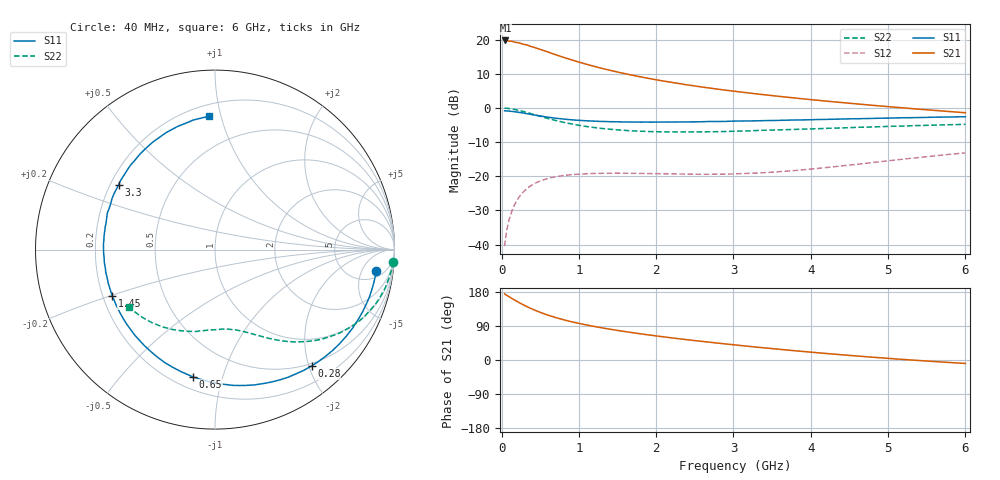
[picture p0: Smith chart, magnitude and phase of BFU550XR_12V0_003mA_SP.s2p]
! Filename:  P:\Prog\Test\Noise\ATS_data\Testdata_Net\03 Spar\BFU550XR_APG2013_45_C05_12p0V_003mA_SP_CM01_D.s2p
! Date/Time: Tue 06/Aug/2013 14:38:18
! BFU550XR_APG2013_45_C05_12p0V_1to35mA_SP_CM01_Bias3_R.s2p
! MDIF S-parameter v. bias file
! BFU550XR_APG2013_45_C05_12p0V_1to35mA_SP_CM01
! Date/time Fri Aug 02 14:58:10 2013
! VAR V_out= 12.0010
! VAR I_out= 2.9950
! VAR V_in= 0.7926
! VAR I_in= 0.0257
! Device data file deembeded for feedlines and parallel
! Original file: \03 Spar\BFU550XR_APG2013_45_C05_12p0V_003mA_SP_CM01_R.s2p
! Feed-files: PR006V01_02082013_Feed1.s2p, PR006V01_02082013_Feed2.s2p
! Parallel-file: PR006V01_02082013_Par.s2p
# MHz S MA R 50
!  Freq-MHz  S11-mag  S11-arg  S21-mag  S21-arg  S12-mag  S12-arg  S22-mag  S22-arg
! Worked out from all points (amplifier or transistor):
!   98 points, 40 MHz to 6 GHz, reference 50 ohm
!   highest |S21| = 19.7 dB at 50 MHz (marker M1)
!   |S21| within 3 dB of that: start of sweep to 552.4 MHz
!   unconditionally stable (mu >= 1): 2.794 GHz to 4.426 GHz
!   at 300 MHz: K = 0.13, MSG = 21.4 dB, |S12| = -24.2 dB
!   at 1.6 GHz: K = 0.60, MSG = 14.6 dB, |S12| = -19.1 dB
!   at 6 GHz: K = 0.81, MSG = 5.9 dB, |S12| = -13.2 dB
!   S11 on the Smith chart (normalised r, x): 40 MHz: 7, -10; 280 MHz: 0.46, -2.05; 650 MHz: 0.27, -0.80; 1.45 GHz: 0.24, -0.20; 3.3 GHz: 0.23, +0.29; 6 GHz: 0.28, +0.91
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40  0.9072 -7.6  9.7 174.6  0.009492 83.8  0.9928 -4.0
50  0.9053 -9.4  9.702 172.6  0.01185 83.3  0.9924 -5.1
120  0.8927 -22.7  9.484 164.2  0.02791 76.2  0.9725 -12.6
180  0.8762 -33.5  9.144 157.0  0.0406 70.2  0.9452 -18.6
240  0.8559 -44.0  8.877 150.1  0.05189 64.7  0.913 -24.0
280  0.8424 -50.3  8.549 145.9  0.05866 61.2  0.889 -27.4
320  0.8257 -57.2  8.391 141.7  0.0647 58.0  0.8628 -30.5
440  0.7823 -74.7  7.575 130.7  0.0796 49.6  0.789 -38.6
550  0.7464 -88.9  6.883 122.0  0.08916 43.2  0.7251 -44.9
650  0.7199 -99.8  6.27 115.2  0.09583 38.6  0.6778 -49.4
850  0.6785 -118.7  5.282 103.7  0.1041 31.5  0.5997 -56.6
1050  0.6531 -133.3  4.511 94.5  0.108 26.7  0.5445 -62.3
1250  0.6367 -145.5  3.917 86.6  0.1104 23.2  0.5086 -66.8
1450  0.6281 -155.7  3.451 79.7  0.1108 20.9  0.4824 -71.0
1750  0.6211 -168.6  2.919 70.5  0.1102 18.9  0.4589 -76.6
2050  0.621 -179.3  2.521 62.3  0.1087 18.6  0.447 -81.9
2500  0.6244 166.7  2.092 51.2  0.1072 20.1  0.4461 -89.4
3100  0.6431 150.8  1.707 38.1  0.1093 25.8  0.4584 -99.2
3300  0.6472 146.0  1.604 33.9  0.1114 27.8  0.4671 -102.5
4100  0.6763 128.3  1.29 18.9  0.1308 35.3  0.4971 -115.6
5200  0.7174 106.8  1.001 1.4  0.1784 37.6  0.5436 -133.3
6000  0.7432 92.8  0.8501 -9.1  0.2198 34.2  0.5752 -145.9
